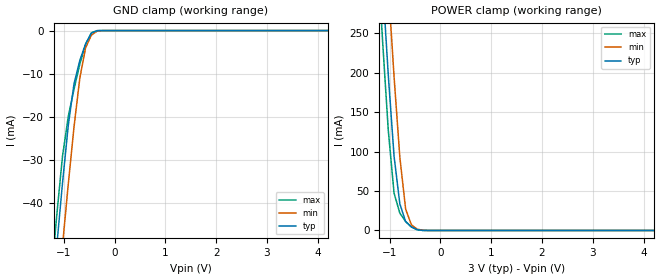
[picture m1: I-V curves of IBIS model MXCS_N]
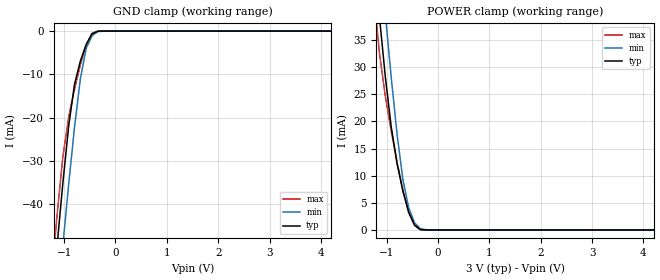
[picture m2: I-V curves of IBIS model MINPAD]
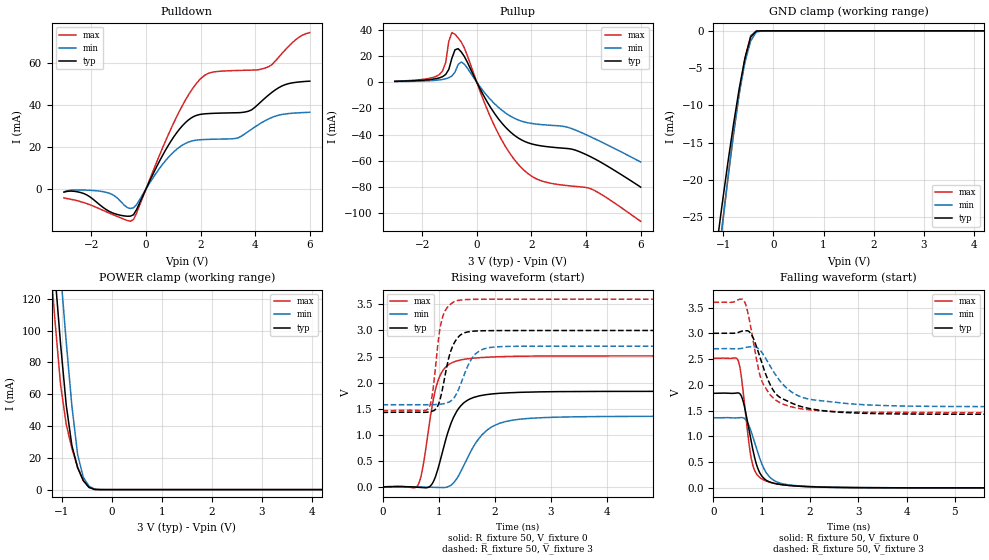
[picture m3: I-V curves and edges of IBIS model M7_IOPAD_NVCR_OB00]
| Created by SiliconSmart  O-2018.09-SP2-3
[IBIS Ver]   4.0
[File Name]   as3a04wa_rev1p4.ibs
[File Rev]   1.4
[Date]   Thursday Mar 21 2024
|[Source]   Avalanche Team
|[Notes]   Generated IBIS models from Silicon Smart
|[Rev 1.0]  Initial Release based on extracted netlist
|   Characterization
|[Rev 1.1]  Update the drive strength table for 3V
|[Rev 1.2]  Recharacterization of MIOPAD with Hspice run in high accuracy mode
|[Rev 1.3]  Recharacterization with Hspice to align with datasheet parameters
|[Rev 1.4]  Update the pin to the package pinout assignment
|[Disclaimer]   THE MODEL LIBRARIES ARE PROVIDED AS IS.
|[Copyright]   Copyright 2019, Avalanche Technology., All Rights Reserved
[Component]   AS30xxA04_WSON
[Manufacturer] Avalanche Technology
| CONTENT :
| This file contains IBIS MODEL for PSRAM device
| AS3016A04
| USAGE :
| The models are derived for the 2.7V to 3.6V I/O Operation.
| Temperatures for model generation: typ: 25, max: -40, min: 125
| Voltages : typ: 3.0V, min: 2.7V, max: 3.6V
| PACKAGES SUPPORTED :
| 8-pad WSON (5.0mm x 6.0mm)
| VERIFICATION
| Errors  : 0
| Warnings: 30
| All warnings due to non-monotonic data:
[Package]
|variable   typ   min   max
R_pkg   8.90E-04   8.89E-04  8.91E-04
L_pkg   1.185E-09  1.18E-09  1.19E-09
C_pkg   2.30E-13   2.21E-13  2.39E-13
[Pin]   signal_name   model_name   R_pin   L_pin   C_pin
1   CS#   MXCS_N   1.05E-01  1.35E-09  9.16E-14
2   SO   MIOPAD   1.05E-01  1.35E-09  9.16E-14
3   WP#   MIOPAD   1.05E-01  1.35E-09  9.16E-14
5   SI   MIOPAD   3.75E-02  3.89E-10  4.24E-14
6   CLK   MINPAD   3.75E-02  3.89E-10  4.24E-14
7   IO_3   MIOPAD   3.75E-02  3.89E-10  4.24E-14
4   VSS   GND   NA   NA   NA
8   VCC   POWER   NA   NA   NA
[Model Selector] MIOPAD
| Model Description
M0_IOPAD_NVCR_OB07   15 Ohms drv strength
M1_IOPAD_NVCR_OB06   20 Ohms drv strength
M2_IOPAD_NVCR_OB05   40 Ohms drv strength
M3_IOPAD_NVCR_OB04   35 Ohms drv strength
M4_IOPAD_NVCR_OB03   45 Ohms drv strength
M5_IOPAD_NVCR_OB02   60 Ohms drv strength
M6_IOPAD_NVCR_OB01   75 Ohms drv strength
M7_IOPAD_NVCR_OB00   35 Ohms drv strength
| Models and submodels in the file (10): MXCS_N (Input), MINPAD (Input), M7_IOPAD_NVCR_OB00 (I/O), M3_IOPAD_NVCR_OB04 (I/O), M5_IOPAD_NVCR_OB02 (I/O), M1_IOPAD_NVCR_OB06 (I/O), M6_IOPAD_NVCR_OB01 (I/O), M2_IOPAD_NVCR_OB05 (I/O), M4_IOPAD_NVCR_OB03 (I/O), M0_IOPAD_NVCR_OB07 (I/O)
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| XCS_N
[Model] MXCS_N
Model_type Input
Enable   Active-High
Vinl  =  0.9
Vinh  =  2.1
| Capacitance  typ   min   max
C_comp   3.070316e-12   2.808436e-12   3.362778e-12
| Variables   typ   min   max
[GND Clamp Reference]   0   0   0
[POWER Clamp Reference]   3   2.7   3.6
[Pulldown Reference]   0   0   0
[Pullup Reference]   3   2.7   3.6
[Temperature Range]   25   125   -40
[Voltage Range]   3   2.7   3.6
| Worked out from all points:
|   GND clamp passes 1 mA (typ) near -0.47 V on its own axis
|   POWER clamp passes 1 mA (typ) near -0.45 V on its own axis
[GND Clamp]
| Voltage   I(typ)   I(min)   I(max)
-3V       -315.1mA   -324.4mA   -312.6mA
-1.252V   -65.4mA    -79.81mA   -58.19mA
-1.138V   -50.1mA    -64.67mA   -42.93mA
-1.024V   -35.38mA   -49.87mA   -29.17mA
-910.3mV  -22.01mA   -35.59mA   -19.91mA
-796.6mV  -12.29mA   -22.27mA   -13.52mA
-682.8mV  -6.93mA    -11.01mA   -7.783mA
-569mV    -3.073mA   -3.973mA   -3.169mA
-455.2mV  -632.4uA   -1.053mA   -499.8uA
-341.4mV  -24.5uA    -114.6uA   -7.616uA
-227.6mV  -421.5nA   -6.331uA   -35.99nA
6V        0A         0A         0A
[POWER Clamp]
| Voltage   I(typ)   I(min)   I(max)
-3V       2.46A      2.566A     2.395A
-1.252V   439.5mA    555.7mA    366.4mA
-1.138V   315.5mA    431.5mA    242.2mA
-1.024V   197.2mA    310.6mA    127mA
-910.3mV  94.22mA    195mA      47.4mA
-796.6mV  33.73mA    92.87mA    21.95mA
-682.8mV  11.27mA    27.26mA    11.43mA
-569mV    4.378mA    7.114mA    4.484mA
-455.2mV  1.088mA    1.626mA    987.1uA
-227.6mV  835.3nA    15.42uA    241.1nA
6V        0A         0A         0A
| INPAD
[Model] MINPAD
Model_type Input
Enable   Active-High
Vinl  =  0.9
Vinh  =  2.1
| Capacitance  typ   min   max
C_comp   2.706389e-12   2.515315e-12   2.924555e-12
| Variables   typ   min   max
[GND Clamp Reference]   0   0   0
[POWER Clamp Reference]   3   2.7   3.6
[Pulldown Reference]   0   0   0
[Pullup Reference]   3   2.7   3.6
[Temperature Range]   25   125   -40
[Voltage Range]   3   2.7   3.6
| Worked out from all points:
|   GND clamp passes 1 mA (typ) near -0.47 V on its own axis
|   POWER clamp passes 1 mA (typ) near -0.46 V on its own axis
[GND Clamp]
| Voltage   I(typ)   I(min)   I(max)
-3V       -312.9mA   -321.9mA   -311mA
-1.252V   -64.97mA   -79.25mA   -57.87mA
-1.138V   -49.77mA   -64.22mA   -42.7mA
-1.024V   -35.15mA   -49.53mA   -29.02mA
-910.3mV  -21.89mA   -35.36mA   -19.81mA
-796.6mV  -12.24mA   -22.14mA   -13.45mA
-682.8mV  -6.904mA   -10.96mA   -7.747mA
-569mV    -3.064mA   -3.962mA   -3.158mA
-455.2mV  -631.5uA   -1.051mA   -499.1uA
-341.4mV  -24.5uA    -114.6uA   -7.616uA
-227.6mV  -421.5nA   -6.331uA   -35.99nA
6V        0A         0A         0A
[POWER Clamp]
| Voltage   I(typ)   I(min)   I(max)
-3V       249.7mA    262.4mA    242mA
-1.252V   50.97mA    63.85mA    43.36mA
-1.138V   39.14mA    51.62mA    32.5mA
-1.024V   28.15mA    39.68mA    24.58mA
-910.3mV  19.01mA    28.18mA    18.3mA
-796.6mV  12.24mA    17.66mA    12.48mA
-682.8mV  7.193mA    9.273mA    7.285mA
-569mV    3.26mA     4.081mA    3.179mA
-455.2mV  915uA      1.304mA    809.1uA
-341.4mV  55.3uA     253.9uA    44.86uA
-113.8mV  7.997nA    700.3nA    881.5pA
6V        0A         0A         0A
[Model] M7_IOPAD_NVCR_OB00
Model_type I/O
Enable   Active-High
Vinl  =  0.9
Vinh  =  2.1
Vmeas =  1.5
Cref  =  30e-12
| Capacitance  typ   min   max
C_comp   3.872127e-12   3.590660e-12   4.190515e-12
| Variables   typ   min   max
[GND Clamp Reference]   0   0   0
[POWER Clamp Reference]   3   2.7   3.6
[Pulldown Reference]   0   0   0
[Pullup Reference]   3   2.7   3.6
[Temperature Range]   25   125   -40
[Voltage Range]   3   2.7   3.6
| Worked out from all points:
|   slope of the pulldown table from 0 to 0.45 V, typ, clamps not added: 37.1 ohm
|   slope of the pullup table from 0 to 0.45 V, typ, clamps not added: 25.9 ohm
|   GND clamp passes 1 mA (typ) near -0.46 V on its own axis
|   POWER clamp passes 1 mA (typ) near -0.42 V on its own axis
|   falling waveform, R_fixture 50, V_fixture 0: 20-80 % time 256ps typ, 326ps min, 201ps max; typ from 1.83 V to 0 V
|   falling waveform, R_fixture 50, V_fixture 3: 20-80 % time 490ps typ, 623ps min, 350ps max; typ from 3 V to 1.43 V
|   rising waveform, R_fixture 50, V_fixture 0: 20-80 % time 339ps typ, 474ps min, 243ps max; typ from 0 V to 1.83 V
|   rising waveform, R_fixture 50, V_fixture 3: 20-80 % time 204ps typ, 275ps min, 147ps max; typ from 1.43 V to 3 V
[GND Clamp]
| Voltage   I(typ)   I(min)   I(max)
-3V       -145.9mA   -153.7mA   -144.2mA
-1.138V   -29.07mA   -33.2mA    -32.68mA
-1.024V   -23.24mA   -26.38mA   -26.15mA
-910.3mV  -17.69mA   -19.83mA   -19.83mA
-796.6mV  -12.47mA   -13.74mA   -13.82mA
-682.8mV  -7.718mA   -8.413mA   -8.316mA
-569mV    -3.663mA   -4.215mA   -3.675mA
-455.2mV  -839.2uA   -1.36mA    -666.1uA
-341.4mV  -35.63uA   -163.9uA   -11.17uA
-113.8mV  -8.642nA   -411.9nA   -1.888nA
6V        0A         0A         0A
[POWER Clamp]
| Voltage   I(typ)   I(min)   I(max)
-3V       949.8mA    993.3mA    923.5mA
-1.252V   183.6mA    231.1mA    154mA
-1.138V   136.7mA    183.8mA    107.6mA
-1.024V   92.09mA    137.6mA    66.35mA
-910.3mV  53.33mA    93.06mA    41.06mA
-796.6mV  27.72mA    52.58mA    25.94mA
-682.8mV  13.75mA    22.15mA    14.29mA
-569mV    5.664mA    7.785mA    5.738mA
-455.2mV  1.446mA    2.116mA    1.305mA
-341.4mV  77.09uA    373.9uA    62.73uA
-227.6mV  1.148uA    21.11uA    332nA
6V        0A         0A         0A
[Pulldown]
| Voltage   I(typ)   I(min)   I(max)
-3V       -1.433mA   -1.306mA   -4.157mA
-2.276V   -2.108mA   -451.4uA   -6.425mA
-1.479V   -9.535mA   -1.453mA   -10.63mA
-455.2mV  -12.21mA   -8.895mA   -14.49mA
931mV     23.15mA    16.61mA    29.13mA
1.448V    31.69mA    21.77mA    42.45mA
1.966V    35.52mA    23.49mA    52.07mA
2.483V    36.1mA     23.77mA    55.8mA
3.745V    37.06mA    27.41mA    56.63mA
4.49V     44.79mA    33.42mA    58.29mA
5.11V     49.81mA    35.81mA    66.46mA
6V        51.42mA    36.59mA    74.56mA
[Pullup]
| Voltage   I(typ)   I(min)   I(max)
-3V       653.5uA    465.2uA    766.8uA
-1.366V   3.311mA    1.742mA    5.899mA
-1.138V   5.906mA    2.581mA    14.98mA
-1.024V   9.73mA     3.378mA    31.24mA
-910.3mV  18.3mA     4.722mA    37.88mA
-796.6mV  24.73mA    7.691mA    36.53mA
-455.2mV  19.63mA    13.8mA     26.19mA
620.7mV   -22.92mA   -15.8mA    -32.1mA
1.655V    -44.22mA   -29.83mA   -65.72mA
2.379V    -48.66mA   -32.38mA   -75.39mA
3.745V    -52.9mA    -37.67mA   -79.8mA
6V        -80.07mA   -60.91mA   -106.2mA
[Ramp]
dV/dt_r   1.10101/0.339017n  0.814816/0.474352n  1.50845/0.242789n
dV/dt_f   0.94313/0.490001n  0.674772/0.62293n  1.28285/0.34977n
R_load = 50
[Falling Waveform]
R_fixture = 50
V_fixture = 0
V_fixture_min = 0
V_fixture_max = 0
| Time   V(typ)   V(min)   V(max)
0s        1.835V     1.358V     2.514V
508.1ps   1.842V     1.359V     2.484V
563ps     1.81V      1.364V     2.266V
628.4ps   1.639V     1.356V     1.772V
754.2ps   1.042V     1.168V     742mV
850.8ps   600.9mV    893.8mV    345.7mV
956.7ps   299.5mV    582.8mV    204.1mV
1.113ns   137.2mV    268.9mV    125.8mV
1.514ns   51.15mV    64.98mV    51.11mV
21.88ns   622.8nV    1.219uV    10.89uV
[Falling Waveform]
R_fixture = 50
V_fixture = 3
V_fixture_min = 2.7
V_fixture_max = 3.6
| Time   V(typ)   V(min)   V(max)
0s        3V         2.7V       3.6V
624.2ps   3.048V     2.716V     3.642V
788.3ps   2.977V     2.74V      3.046V
963.4ps   2.539V     2.676V     2.19V
1.115ns   2.134V     2.463V     1.888V
1.348ns   1.775V     2.113V     1.67V
1.624ns   1.645V     1.858V     1.571V
2.036ns   1.53V      1.713V     1.509V
4.44ns    1.431V     1.582V     1.463V
21.88ns   1.428V     1.575V     1.462V
[Rising Waveform]
R_fixture = 50
V_fixture = 0
V_fixture_min = 0
V_fixture_max = 0
| Time   V(typ)   V(min)   V(max)
0s        414.5nV    971.2nV    10.8uV
619.8ps   -611.3uV   5.171mV    21.45mV
717.4ps   -8.991mV   2.855mV    378.7mV
871ps     45.71mV    -2.403mV   1.477V
1.013ns   453.4mV    -7.701mV   2.11V
1.262ns   1.331V     79.29mV    2.395V
1.571ns   1.696V     685.2mV    2.465V
2.049ns   1.795V     1.209V     2.497V
3.034ns   1.828V     1.339V     2.512V
21.88ns   1.835V     1.358V     2.514V
[Rising Waveform]
R_fixture = 50
V_fixture = 3
V_fixture_min = 2.7
V_fixture_max = 3.6
| Time   V(typ)   V(min)   V(max)
0s        1.428V     1.575V     1.462V
810.7ps   1.438V     1.579V     1.497V
887.5ps   1.456V     1.579V     1.779V
1.003ns   1.607V     1.585V     2.894V
1.068ns   1.883V     1.594V     3.253V
1.21ns    2.592V     1.647V     3.502V
1.401ns   2.923V     2.001V     3.585V
1.655ns   2.99V      2.55V      3.596V
2.116ns   2.998V     2.692V     3.599V
21.88ns   3V         2.7V       3.6V
